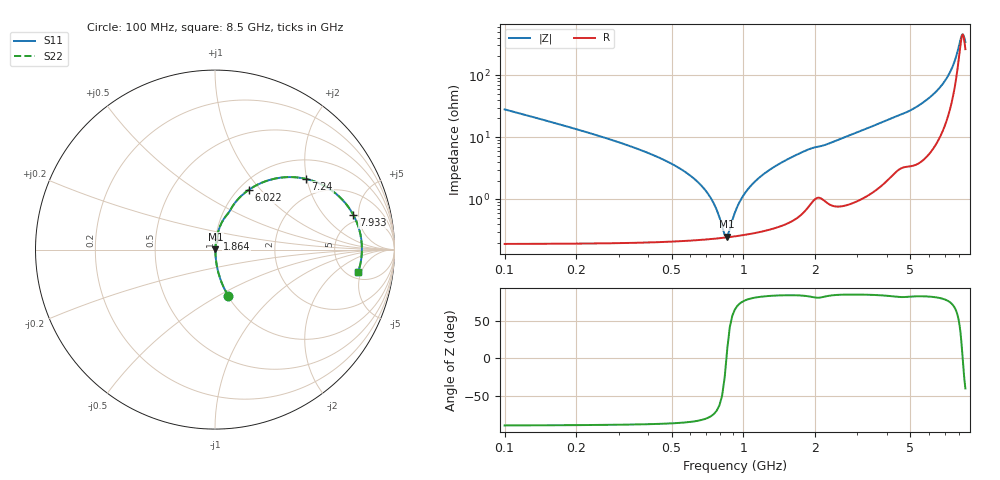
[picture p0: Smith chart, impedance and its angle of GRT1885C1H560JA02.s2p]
!Murata Part Number: GRT1885C1H560JA02
!These Parameters are Measured in Series Mode Connection
!Data Generated on Jun 19, 2026
!  o--ll--o
!Port1  Port2
!  o------o
!Operation Temp=25[degC], DC Bias Voltage=0[V]
!Freq. Start=100[MHz] Stop=9[GHz] 401[Steps]
# Hz S RI R 50
!Freq.(Hz) S11(Real) S11(Imag) S21(Real) S21(Imag) S12(Real) S12(Imag) S22(Real) S22(Imag)
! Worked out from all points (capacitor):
!   401 points, 100 MHz to 8.5 GHz, reference 50 ohm
!   read as one part in series: C = 56 pF near 142 MHz
!   lowest |Z| = 250 mohm at 856 MHz (marker M1)
!   series resonance near 848.8 MHz, so ESL is about 630 pH
!   S11 on the Smith chart (normalised r, x): 100 MHz: 1.00, -0.56; 1.864 GHz: 1.01, +0.13; 6.022 GHz: 1.11, +0.87; 7.24 GHz: 1.48, +1.98; 7.933 GHz: 4.08, +4.29; 8.5 GHz: 6.23, -4.40
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1e8  0.0744 -0.259  0.9256 0.259  0.9256 0.259  0.0744 -0.259
2.89e8  0.00943 -0.0861  0.9906 0.0861  0.9906 0.0861  0.00943 -0.0861
6.46e8  0.00254 -0.0185  0.9975 0.0185  0.9975 0.0185  0.00254 -0.0185
7.3e8  0.00238 -0.0102  0.9976 0.0102  0.9976 0.0102  0.00238 -0.0102
8.14e8  0.00238 -0.00282  0.9976 0.00282  0.9976 0.00282  0.00238 -0.00282
8.56e8  0.00243 0.000577  0.9976 -0.000577  0.9976 -0.000577  0.00243 0.000577
8.77e8  0.00246 0.00221  0.9975 -0.00221  0.9975 -0.00221  0.00246 0.00221
9.82e8  0.00271 0.00992  0.9973 -0.00992  0.9973 -0.00992  0.00271 0.00992
1.087e9  0.00308 0.017  0.9969 -0.017  0.9969 -0.017  0.00308 0.017
1.255e9  0.0039 0.0275  0.9961 -0.0275  0.9961 -0.0275  0.0039 0.0275
1.507e9  0.00573 0.0421  0.9943 -0.0421  0.9943 -0.0421  0.00573 0.0421
1.864e9  0.0111 0.0614  0.9889 -0.0614  0.9889 -0.0614  0.0111 0.0614
2.914e9  0.0215 0.1114  0.9785 -0.1114  0.9785 -0.1114  0.0215 0.1114
4.3e9  0.0648 0.1913  0.9352 -0.1913  0.9352 -0.1913  0.0648 0.1913
5.707e9  0.1484 0.301  0.8516 -0.301  0.8516 -0.301  0.1484 0.301
6.022e9  0.1885 0.333  0.8115 -0.333  0.8115 -0.333  0.1885 0.333
7.114e9  0.459 0.4019  0.541 -0.4019  0.541 -0.4019  0.459 0.4019
7.24e9  0.507 0.3939  0.493 -0.3939  0.493 -0.3939  0.507 0.3939
7.618e9  0.6609 0.3217  0.3391 -0.3217  0.3391 -0.3217  0.6609 0.3217
7.933e9  0.7702 0.194  0.2298 -0.194  0.2298 -0.194  0.7702 0.194
8.248e9  0.8183 0.0193  0.1817 -0.0193  0.1817 -0.0193  0.8183 0.0193
8.5e9  0.7982 -0.1229  0.2018 0.1229  0.2018 0.1229  0.7982 -0.1229
